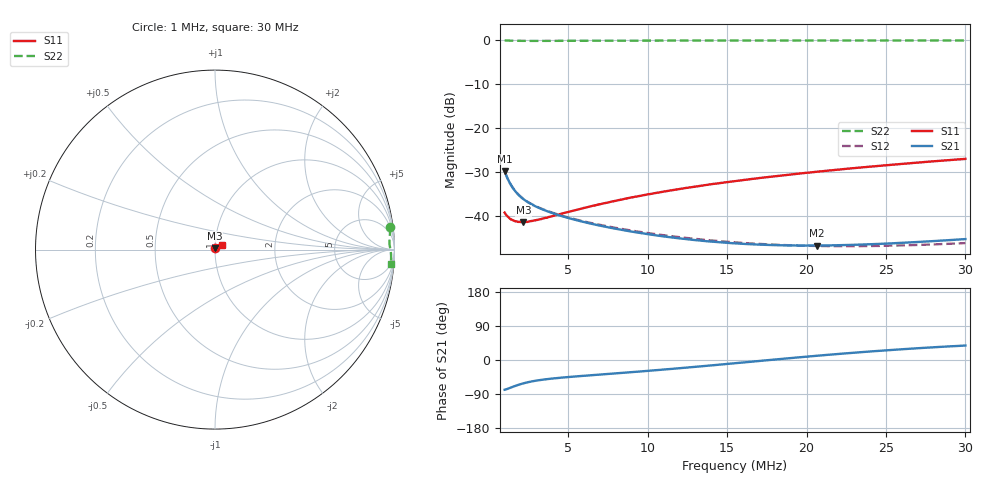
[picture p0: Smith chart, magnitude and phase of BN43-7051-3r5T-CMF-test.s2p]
! ListType=Log
!!Balun BN43-7051 3.5T test
# MHZ S RI R 50
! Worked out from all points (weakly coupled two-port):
!   101 points, 1 MHz to 30 MHz, reference 50 ohm
!   highest |S21| = -29.75 dB at 1 MHz (marker M1); lowest = -46.6 dB at 20.64 MHz (marker M2)
!   lowest |S11| = -41.3 dB at 2.186 MHz (marker M3), VSWR 1.02, Z = 49.9 + j0.846 ohm
!   |S11| at or under -10 dB: start of sweep to end of sweep
!   |S22| runs from -0.2 to -0.1 dB; largest |S21 - S12| = 0.00094
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1  -0.00219 0.0108  0.0065 -0.0319  0.00658 -0.0319  0.9756 0.1253
1.107423  -0.002 0.0101  0.00641 -0.0283  0.0065 -0.0282  0.976 0.1106
1.226386  -0.00197 0.00959  0.00651 -0.0251  0.00658 -0.0251  0.9756 0.0977
1.405116  -0.0018 0.00902  0.00676 -0.0215  0.00683 -0.0215  0.9746 0.0831
1.504023  -0.00178 0.00887  0.0069 -0.02  0.00696 -0.02  0.9741 0.0768
1.66559  -0.00172 0.0086  0.00708 -0.018  0.00714 -0.018  0.9734 0.0683
1.844513  -0.00163 0.00848  0.00725 -0.0162  0.0073 -0.0162  0.9726 0.0609
2.186442  -0.00132 0.00848  0.00743 -0.0138  0.00748 -0.0138  0.9719 0.0503
2.421316  -0.0012 0.00853  0.0075 -0.0125  0.00754 -0.0126  0.9717 0.045
2.774191  -0.000892 0.00883  0.0075 -0.0111  0.00754 -0.0112  0.9716 0.0386
3.519937  -0.000242 0.00954  0.00732 -0.00913  0.00735 -0.00922  0.9723 0.0289
4.620666  0.000757 0.0107  0.00691 -0.00726  0.00695 -0.00739  0.974 0.0189
5.862773  0.00194 0.0121  0.00648 -0.00585  0.00651 -0.00601  0.9758 0.0104
7.9624  0.00403 0.0144  0.0059 -0.00418  0.00595 -0.00441  0.9779 -0.000938
10.81396  0.00716 0.0173  0.00538 -0.00261  0.00543 -0.00292  0.9797 -0.0136
12.81861  0.00959 0.0192  0.00512 -0.00173  0.00517 -0.00211  0.9804 -0.0217
15.72057  0.0134 0.0214  0.00486 -0.000654  0.0049 -0.00113  0.981 -0.0324
18.01163  0.0168 0.0229  0.00471 0.000103  0.00475 -0.00044  0.9812 -0.0406
20.63659  0.0209 0.0242  0.00457 0.000896  0.0046 0.000267  0.9811 -0.0496
22.85344  0.0246 0.0249  0.00449 0.00152  0.00451 0.000823  0.981 -0.0571
25.30843  0.0288 0.0252  0.00442 0.00219  0.00443 0.00141  0.9806 -0.0651
30  0.0374 0.0245  0.00434 0.0034  0.00431 0.00247  0.9796 -0.0803
